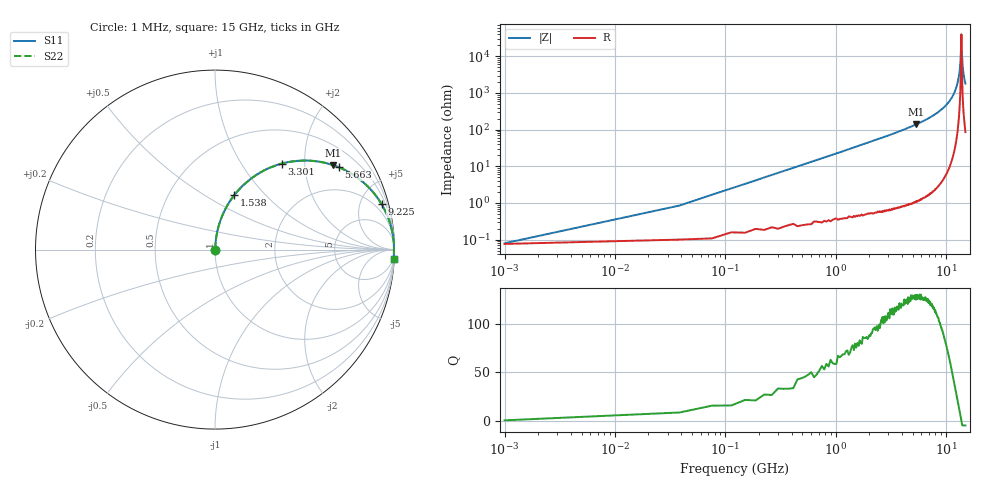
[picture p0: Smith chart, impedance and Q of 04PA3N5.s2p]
! Coilcraft 0402PA-3N5 Chip Inductor
! 11 March 2004
# MHZ S MA R 50
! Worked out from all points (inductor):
!   401 points, 1 MHz to 15 GHz, reference 50 ohm
!   read as one part in series: L = 3.5 nH near 76 MHz
!   highest Q = 130 at 5.363 GHz (marker M1), where L = 4.12 nH
!   self-resonance near 13.8 GHz
!   S11 on the Smith chart (normalised r, x): 1 MHz: 1.00, +0.00; 1.538 GHz: 1.01, +0.69; 3.301 GHz: 1.01, +1.54; 5.663 GHz: 1.02, +3.00; 9.225 GHz: 1.08, +7.33; 15 GHz: 3, -36
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1  0.0005723 22.6  0.999 -0.0  0.999 -0.0  0.0005723 22.6
113.492  0.025 85.2  0.998 -1.4  0.998 -1.4  0.025 85.2
188.487  0.041 85.2  0.997 -2.4  0.997 -2.4  0.041 85.2
300.98  0.066 84.4  0.996 -3.8  0.996 -3.8  0.066 84.4
750.95  0.163 79.5  0.984 -9.4  0.984 -9.4  0.163 79.5
1538.397  0.323 70.4  0.942 -18.8  0.942 -18.8  0.323 70.4
2513.332  0.494 59.8  0.864 -29.6  0.864 -29.6  0.494 59.8
3300.78  0.607 52.1  0.789 -37.4  0.789 -37.4  0.607 52.1
5025.665  0.784 38.0  0.615 -51.6  0.615 -51.6  0.784 38.0
5363.143  0.809 35.6  0.582 -54.0  0.582 -54.0  0.809 35.6
5663.123  0.829 33.6  0.553 -56.0  0.553 -56.0  0.829 33.6
7500.5  0.917 23.1  0.392 -66.5  0.392 -66.5  0.917 23.1
9225.385  0.962 15.2  0.262 -74.2  0.262 -74.2  0.962 15.2
10012.83  0.975 12.1  0.21 -77.2  0.21 -77.2  0.975 12.1
12525.17  0.995 3.7  0.064 -84.1  0.064 -84.1  0.995 3.7
13350.11  0.997 1.2  0.022 -82.2  0.022 -82.2  0.997 1.2
13575.09  0.997 0.6  0.011 -76.3  0.011 -76.3  0.997 0.6
13800.08  0.997 0.0  0.002523 -0.4  0.002523 -0.4  0.997 0.0
13875.08  0.997 -0.2  0.004352 54.3  0.004352 54.3  0.997 -0.2
14025.07  0.997 -0.6  0.011 76.0  0.011 76.0  0.997 -0.6
14250.05  0.997 -1.2  0.021 81.9  0.021 81.9  0.997 -1.2
15000  0.996 -3.1  0.055 84.1  0.055 84.1  0.996 -3.1
